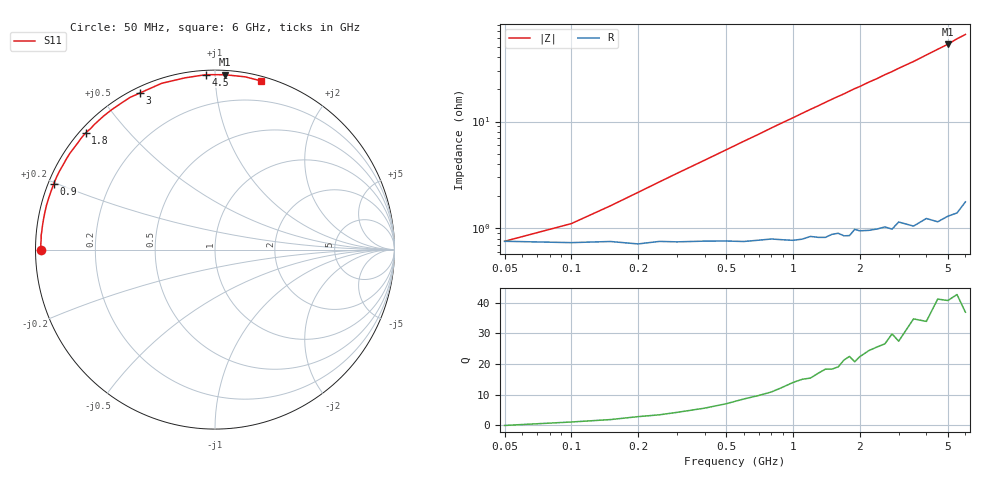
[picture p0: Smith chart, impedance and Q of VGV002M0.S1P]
! Infineon Technologies  Discrete & RF Semiconductors
! BB 831
! Si Tuning Diode in SOD323
! VR =
! S-Parameters:  July  1999
# GHz  S  MA  R  50
!  f  S11
! GHz  MAG  ANG
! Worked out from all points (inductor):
!   34 points, 50 MHz to 6 GHz, reference 50 ohm
!   read as one part to ground: L = 1.69 nH near 250 MHz
!   highest Q = 41.1 at 5 GHz (marker M1), where L = 1.68 nH
!   S11 on the Smith chart (normalised r, x): 50 MHz: 0.02, +0.00; 900 MHz: 0.02, +0.20; 1.8 GHz: 0.02, +0.38; 3 GHz: 0.02, +0.63; 4.5 GHz: 0.02, +0.95; 6 GHz: 0.04, +1.30
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0.05  0.9701 180.0
0.1  0.971 178.1
0.2  0.9718 175.3
0.3  0.9706 172.7
0.5  0.9703 167.7
0.6  0.9708 165.2
0.8  0.9696 160.3
0.9  0.9703 157.9
1  0.9709 155.6
1.1  0.9704 153.2
1.3  0.9699 148.7
1.4  0.9702 146.4
1.6  0.9683 142.1
1.7  0.9703 140.1
1.8  0.9706 137.9
1.9  0.9669 135.8
2  0.9683 134.0
2.2  0.969 129.9
2.4  0.969 126.4
2.6  0.9688 122.5
2.8  0.9711 119.2
3  0.9677 115.6
3.5  0.9729 107.8
4  0.9714 100.0
4.5  0.976 93.0
5  0.9758 86.8
5.5  0.9771 80.1
6  0.9742 74.9
